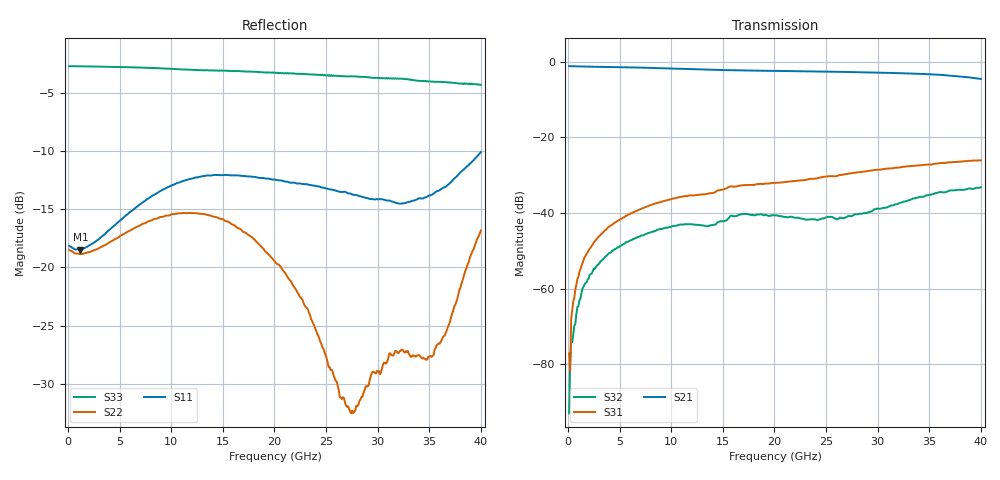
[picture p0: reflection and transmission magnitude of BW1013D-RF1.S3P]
!  3-Port S-parameters saved by WinCal
! VAR MeasName=S-Parameters (CALIBRATED_DATA) read from VNA (N5245A)
! VAR MeasDate=12/26/2016 18:41:11
! VAR NAME=158306_25-RF1
! VAR FILENAME=158306_25-RF1.S3P
! VAR DATE=12/26/2016 18:41:11
! VAR PHYS_PORTS=1,2,3
# Hz S RI R 50
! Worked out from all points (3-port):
!   401 points, 100 MHz to 40 GHz, reference 50 ohm
!   strongest paths, dB at 100 MHz, 10.07 GHz, 20.05 GHz, 30.02 GHz, 40 GHz:
!     S21: -1.2, -1.8, -2.4, -2.8, -4.5
!     S31: -77.1, -36.2, -32.0, -28.5, -26.0
!     S32: -93.0, -43.5, -40.6, -38.8, -33.2
!   lowest |S11| = -18.5 dB at 1.197 GHz (marker M1), VSWR 1.27, Z = 62.2 - j5.56 ohm
!   |S11| at or under -10 dB: start of sweep to end of sweep
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1e8  0.1237 -0.00546  0.8758 -0.0113  9.8e-05 -4.94e-05
     0.8758 -0.0113  0.1188 -0.0047  -2.7e-05 -1.19e-05
     0.000111 8.54e-05  2.23e-05 2.98e-06  -0.731 0.00273
5.9875e8  0.1174 -0.0255  0.8685 -0.0596  -0.000116 0.000738
          0.8687 -0.0596  0.1133 -0.0218  -0.000102 0.00024
          -0.000159 0.000732  -0.000127 0.000293  -0.7306 0.0155
1.19725e9  0.1107 -0.0441  0.8586 -0.1117  -0.000233 0.00176
           0.8587 -0.1119  0.1076 -0.0379  -0.00023 0.000726
           -0.000209 0.00181  -0.000213 0.000707  -0.7295 0.0313
3.0925e9  0.0895 -0.0995  0.8143 -0.269  0.000805 0.00503
          0.8141 -0.2691  0.087 -0.085  0.000385 0.00222
          0.000838 0.00497  0.00039 0.0022  -0.7232 0.0791
6.484e9  0.0207 -0.1787  0.6661 -0.5134  0.00502 0.00921
         0.6659 -0.5136  0.0207 -0.1466  0.00296 0.00359
         0.00501 0.00922  0.00296 0.00356  -0.7032 0.1585
1.296775e10  -0.1506 -0.1948  0.2236 -0.7594  0.0151 0.00902
             0.2233 -0.7594  -0.1189 -0.1214  0.00685 0.000393
             0.0151 0.00904  0.00685 0.0004  -0.6361 0.2977
2.005e10  -0.2223 -0.0851  -0.2792 -0.7051  0.0252 0.00079
          -0.2795 -0.7049  -0.1053 -0.0125  0.0073 -0.00578
          0.0251 0.000798  0.00735 -0.00573  -0.5272 0.4388
2.753125e10  -0.2026 0.0347  -0.6635 -0.3077  0.03 -0.0157
             -0.6638 -0.3069  -0.017 -0.0173  0.00483 -0.00785
             0.03 -0.0156  0.00481 -0.00785  -0.3701 0.5477
3.5212e10  -0.0394 0.2011  -0.6169 0.2916  0.0132 -0.0417
           -0.6169 0.2922  0.0199 -0.0362  -0.00368 -0.0173
           0.0133 -0.0417  -0.0036 -0.0172  -0.1502 0.6091
4e10  0.2525 0.1845  -0.289 0.5182  -0.0138 -0.0477
      -0.2883 0.5186  0.1272 -0.0676  -0.0177 -0.0131
      -0.0137 -0.048  -0.0176 -0.0132  -0.00538 0.608
